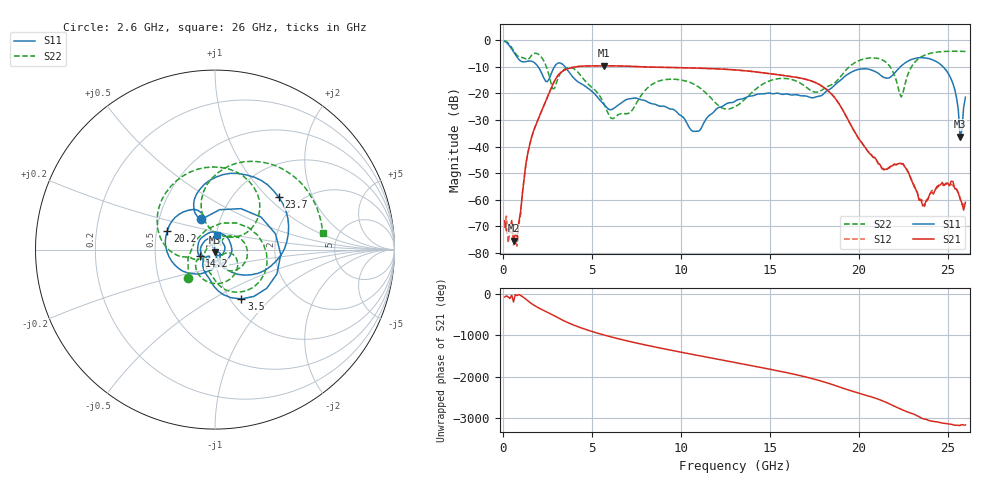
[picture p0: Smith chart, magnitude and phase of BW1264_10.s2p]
!Keysight Technologies,N5245B,MY57181159,A.13.60.06
!Date: Friday, December 18, 2020 23:52:26
!Correction: S11(Full 2 Port(1,2))
!S21(Full 2 Port(1,2))
!S12(Full 2 Port(1,2))
!S22(Full 2 Port(1,2))
!S2P File: Measurements: S11, S21, S12, S22:
# Hz S  dB  R 50
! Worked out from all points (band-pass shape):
!   260 points, 100 MHz to 26 GHz, reference 50 ohm
!   highest |S21| = -9.72 dB at 5.7 GHz (marker M1); lowest = -75.3 dB at 600 MHz (marker M2)
!   |S21| within 3 dB of the highest: 3.182 GHz to 15.06 GHz (11.88 GHz wide, 130 % of centre)
!   lowest |S11| = -36.2 dB at 25.7 GHz (marker M3), VSWR 1.03, Z = 50 - j1.54 ohm
!   |S11| at or under -10 dB: 1.977 GHz to 2.906 GHz (929.5 MHz wide, 38.1 % of centre); 3.484 GHz to 22.36 GHz (18.87 GHz wide, 146 % of centre); 24.73 GHz to end of sweep
!   |S22| runs from -29.5 to -0.2 dB; largest |S21 - S12| = 0.00049
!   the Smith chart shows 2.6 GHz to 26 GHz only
!   S11 on the Smith chart (normalised r, x): 2.6 GHz: 0.81, +0.28; 3.5 GHz: 1.12, -0.69; 14.2 GHz: 0.84, -0.06; 20.2 GHz: 0.57, +0.13; 23.7 GHz: 1.57, +1.17; 26 GHz: 1.01, +0.17
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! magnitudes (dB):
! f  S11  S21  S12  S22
! 100 MHz  -0.5  -67.8  -70.6  -0.2
! 600 MHz  -4.4  -75.3  -76.9  -3.9
! 800 MHz  -6.5  -73.8  -77.4  -5.8
! 1.5 GHz  -7.9  -39.6  -39.6  -6.9
! 2.6 GHz  -14.7  -19.9  -19.9  -13.3
! 3.5 GHz  -10.1  -11.2  -11.2  -10.8
! 4.5 GHz  -16.8  -9.8  -9.8  -14.4
! 5.7 GHz  -24.4  -9.7  -9.7  -24.2
! 7.1 GHz  -22.1  -9.9  -9.9  -27.4
! 8.8 GHz  -24.8  -10.3  -10.3  -15.4
! 10.9 GHz  -34.3  -10.6  -10.6  -17.2
! 13.1 GHz  -22.8  -11.3  -11.3  -24.9
! 14.2 GHz  -20.6  -12.0  -12.0  -18.6
! 17.4 GHz  -21.7  -15.5  -15.5  -19.3
! 20.2 GHz  -10.9  -38.8  -38.9  -7.3
! 21.7 GHz  -14.3  -47.9  -48.1  -9.5
! 22.4 GHz  -9.7  -46.5  -46.3  -21.4
! 23.7 GHz  -6.7  -62.0  -62.5  -5.8
! 25.2 GHz  -14.7  -53.0  -54.2  -4.3
! 25.5 GHz  -21.6  -56.0  -56.0  -4.3
! 25.7 GHz  -36.2  -59.6  -59.3  -4.3
! 26 GHz  -21.5  -60.9  -63.1  -4.3
